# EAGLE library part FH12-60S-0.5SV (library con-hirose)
0.5mm and 1mm Pitch Connectors For FPC/FFC Source: Data sheet
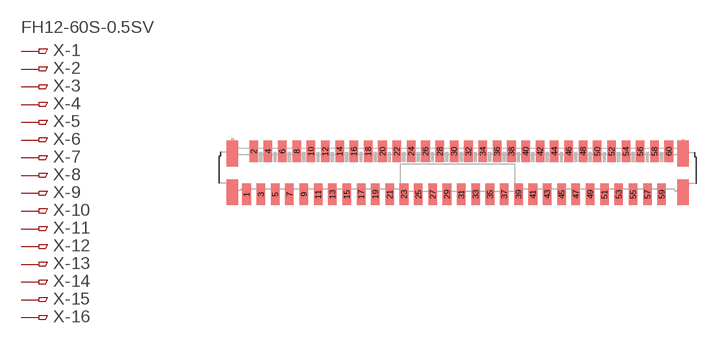
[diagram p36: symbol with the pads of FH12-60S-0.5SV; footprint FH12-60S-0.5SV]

Designator prefix X; gates -1=PINV -2=PIN -3=PIN -4=PIN -5=PIN -6=PIN -7=PIN -8=PIN -9=PIN -10=PIN -11=PIN -12=PIN -13=PIN -14=PIN -15=PIN -16=PIN -17=PIN -18=PIN -19=PIN -20=PIN -21=PIN -22=PIN -23=PIN -24=PIN -25=PIN -26=PIN -27=PIN -28=PIN -29=PIN -30=PIN -31=PIN -32=PIN -33=PIN -34=PIN -35=PIN -36=PIN -37=PIN -38=PIN -39=PIN -40=PIN -41=PIN -42=PIN -43=PIN -44=PIN -45=PIN -46=PIN -47=PIN -48=PIN -49=PIN -50=PIN -51=PIN -52=PIN -53=PIN -54=PIN -55=PIN -56=PIN -57=PIN -58=PIN -59=PIN -60=PIN

## FH12-60S-0.5SV (OC_FARNELL: unknown; OC_NEWARK: unknown)  [FH12-60S-0.5SV]
1  -1:1  pas
2  -2:1  pas
3  -3:1  pas
4  -4:1  pas
5  -5:1  pas
6  -6:1  pas
7  -7:1  pas
8  -8:1  pas
9  -9:1  pas
10  -10:1  pas
11  -11:1  pas
12  -12:1  pas
13  -13:1  pas
14  -14:1  pas
15  -15:1  pas
16  -16:1  pas
17  -17:1  pas
18  -18:1  pas
19  -19:1  pas
20  -20:1  pas
21  -21:1  pas
22  -22:1  pas
23  -23:1  pas
24  -24:1  pas
25  -25:1  pas
26  -26:1  pas
27  -27:1  pas
28  -28:1  pas
29  -29:1  pas
30  -30:1  pas
31  -31:1  pas
32  -32:1  pas
33  -33:1  pas
34  -34:1  pas
35  -35:1  pas
36  -36:1  pas
37  -37:1  pas
38  -38:1  pas
39  -39:1  pas
40  -40:1  pas
41  -41:1  pas
42  -42:1  pas
43  -43:1  pas
44  -44:1  pas
45  -45:1  pas
46  -46:1  pas
47  -47:1  pas
48  -48:1  pas
49  -49:1  pas
50  -50:1  pas
51  -51:1  pas
52  -52:1  pas
53  -53:1  pas
54  -54:1  pas
55  -55:1  pas
56  -56:1  pas
57  -57:1  pas
58  -58:1  pas
59  -59:1  pas
60  -60:1  pas

## Footprint FH12-60S-0.5SV (pad centres in mm)
0.5mm Pitch Connectors For FPC/FFC Source: Data sheet
smd 0.6 x 1.5: 1 -14.75,-1.5; 2 -14.25,1.5; 3 -13.75,-1.5; 4 -13.25,1.5; 5 -12.75,-1.5; 6 -12.25,1.5; 7 -11.75,-1.5; 8 -11.25,1.5; 9 -10.75,-1.5; 10 -10.25,1.5; 11 -9.75,-1.5; 12 -9.25,1.5; 13 -8.75,-1.5; 14 -8.25,1.5; 15 -7.75,-1.5; 16 -7.25,1.5; 17 -6.75,-1.5; 18 -6.25,1.5; 19 -5.75,-1.5; 20 -5.25,1.5; 21 -4.75,-1.5; 22 -4.25,1.5; 23 -3.75,-1.5; 24 -3.25,1.5; 25 -2.75,-1.5; 26 -2.25,1.5; 27 -1.75,-1.5; 28 -1.25,1.5; 29 -0.75,-1.5; 30 -0.25,1.5; 31 0.25,-1.5; 32 0.75,1.5; 33 1.25,-1.5; 34 1.75,1.5; 35 2.25,-1.5; 36 2.75,1.5; 37 3.25,-1.5; 38 3.75,1.5; 39 4.25,-1.5; 40 4.75,1.5; 41 5.25,-1.5; 42 5.75,1.5; 43 6.25,-1.5; 44 6.75,1.5; 45 7.25,-1.5; 46 7.75,1.5; 47 8.25,-1.5; 48 8.75,1.5; 49 9.25,-1.5; 50 9.75,1.5; 51 10.25,-1.5; 52 10.75,1.5; 53 11.25,-1.5; 54 11.75,1.5; 55 12.25,-1.5; 56 12.75,1.5; 57 13.25,-1.5; 58 13.75,1.5; 59 14.25,-1.5; 60 14.75,1.5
